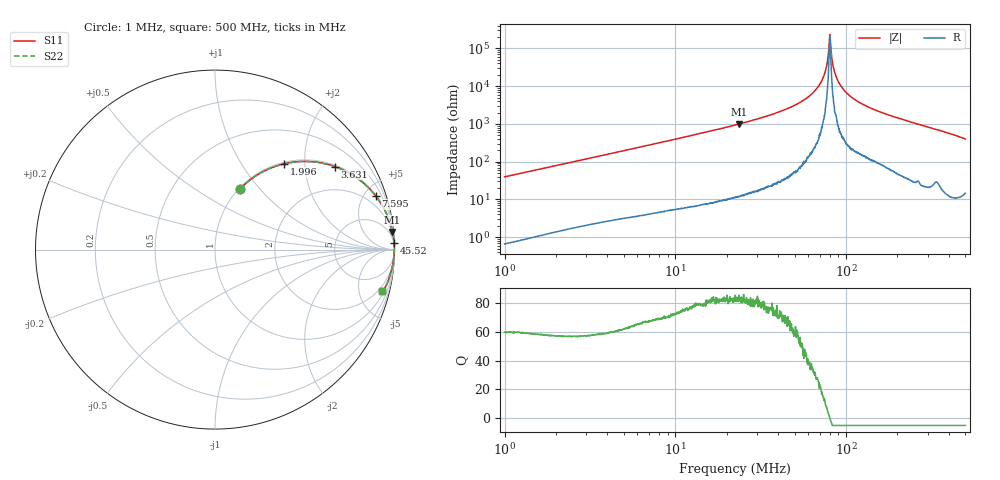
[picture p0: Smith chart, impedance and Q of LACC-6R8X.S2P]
!s-Parameter Generated by FASTRON Sdn. Bhd.
!FASTRON P/N : LACC-6R8X
!Keysight Technologies,E4991B,MY54100416,A.01.15
!Date: Wed Mar 18 09:19:37 2026
!Version  : Rev00 Wed Mar 18 09:19:37 2026
!Data & Calibration Information:
!PortZ  Port1:50+j0  Port2:50+j0
!When reading, reference impedance value at option line is always used.
!Remarks : This data is being provided solely for informational purposes.
!Freq	S11	S21	S12	S22
# Hz S dB R 50
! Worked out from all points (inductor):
!   1601 points, 1 MHz to 500 MHz, reference 50 ohm
!   read as one part in series: L = 6.3 uH near 1.032 MHz
!   highest Q = 83.3 at 23.7 MHz (marker M1), where L = 6.7 uH
!   self-resonance near 80.25 MHz
!   S11 on the Smith chart (normalised r, x): 1 MHz: 1.01, +0.79; 1.996 MHz: 1.03, +1.57; 3.631 MHz: 1.05, +2.85; 7.595 MHz: 1.09, +5.95; 45.52 MHz: 2, +51; 500 MHz: 1.29, -7.96
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1000000  -8.71 67.5  -0.68 -21.5  -0.68 -21.5  -8.71 67.5
1996459  -4.24 51.2  -2.17 -37.8  -2.17 -37.8  -4.24 51.2
2820919  -2.66 41.6  -3.56 -47.4  -3.56 -47.4  -2.66 41.6
3631084  -1.81 34.8  -4.88 -54.2  -4.88 -54.2  -1.81 34.8
7595196  -0.50 18.5  -9.97 -70.7  -9.97 -70.7  -0.50 18.5
7957584  -0.46 17.7  -10.34 -71.5  -10.34 -71.5  -0.46 17.7
2.236068e7  -0.06 6.1  -19.45 -83.2  -19.45 -83.2  -0.06 6.1
2.370216e7  -0.05 5.7  -20.04 -83.6  -20.04 -83.6  -0.05 5.7
4.551764e7  -0.01 2.2  -28.17 -87.0  -28.17 -87.0  -0.01 2.2
6.307767e7  -0.01 0.9  -35.92 -87.5  -35.92 -87.5  -0.01 0.9
6.87047e7  -0.00 0.6  -39.72 -87.2  -39.72 -87.2  -0.00 0.6
7.310989e7  -0.00 0.4  -44.07 -86.0  -44.07 -86.0  -0.00 0.4
7.600545e7  -0.00 0.2  -48.60 -83.6  -48.60 -83.6  -0.00 0.2
7.901568e7  -0.00 0.1  -58.32 -69.4  -58.32 -69.4  -0.00 0.1
8.056521e7  -0.00 -0.0  -67.36 18.2  -67.36 18.2  -0.00 -0.0
8.214513e7  -0.00 -0.1  -56.57 72.4  -56.57 72.4  -0.00 -0.1
8.47377e7  -0.00 -0.2  -49.00 83.1  -49.00 83.1  -0.00 -0.2
8.74121e7  -0.00 -0.3  -45.16 84.3  -45.16 84.3  -0.00 -0.3
9.859709e7  -0.01 -0.8  -37.32 86.5  -37.32 86.5  -0.01 -0.8
1.235099e8  -0.02 -1.7  -30.68 85.8  -30.68 85.8  -0.02 -1.7
1.77937e8  -0.03 -3.3  -24.75 84.6  -24.75 84.6  -0.03 -3.3
5e8  -0.34 -14.0  -12.34 73.9  -12.34 73.9  -0.34 -14.0
